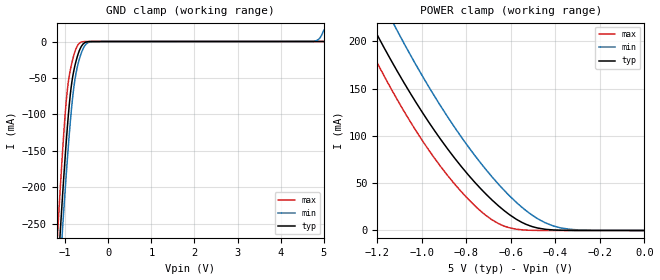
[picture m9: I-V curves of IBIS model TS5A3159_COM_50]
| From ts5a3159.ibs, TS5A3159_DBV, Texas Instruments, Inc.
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[Model]   TS5A3159_COM_50
Model_type  Terminator
| variable   typ   min   max
C_comp   47.33pF   35.67pF   55.52pF
| C_tri-state   47.33pF   35.67pF   55.52pF
[Temperature Range]   40   100   -40
| Ambient temperature   25   85   -40
[Voltage range]   5   4.5   5.5
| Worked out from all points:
|   GND clamp passes 1 mA (typ) near -0.52 V on its own axis
|   POWER clamp passes 1 mA (typ) near -0.43 V on its own axis
[GND Clamp]
| TS5A3159_COM_50
|   Voltage   I(typ)   I(min)   I(max)
-5V       -5.262A    -5.087A    -5.543A
-1.2V     -346.1mA   -388.8mA   -289.8mA
-1.165V   -311.2mA   -354.9mA   -253.3mA
-1.105V   -253.2mA   -298.2mA   -193.3mA
-1.075V   -225.2mA   -270.5mA   -164.7mA
-995mV    -154.6mA   -199.9mA   -96.35mA
-930mV    -104.1mA   -146.9mA   -57.18mA
-795mV    -38.98mA   -61.45mA   -18.02mA
-635mV    -7.878mA   -17.44mA   -1.035mA
-390mV    -30.92uA   -299.6uA   -177.5nA
4.73V     5.259nA    128uA      5.068nA
5V        6.931nA    15.56mA    5.361nA
[POWER Clamp]
| TS5A3159_COM_50
|   Voltage   I(typ)   I(min)   I(max)
-5V       3.29A      3.385A     3.516A
-1.29V    248.4mA    297.3mA    220.1mA
-1.26V    234.3mA    282.2mA    205.5mA
-1.2V     207.1mA    253mA      177.5mA
-1.11V    168.7mA    211.5mA    138.5mA
-940mV    104.9mA    141.2mA    75.69mA
-790mV    58.62mA    88.39mA    32.93mA
-655mV    26.01mA    48.92mA    7.266mA
-530mV    6.362mA    20.74mA    382.3uA
-445mV    1.258mA    8.112mA    23uA
-375mV    233uA      2.688mA    1.591uA
0V        0A         0A         0A
